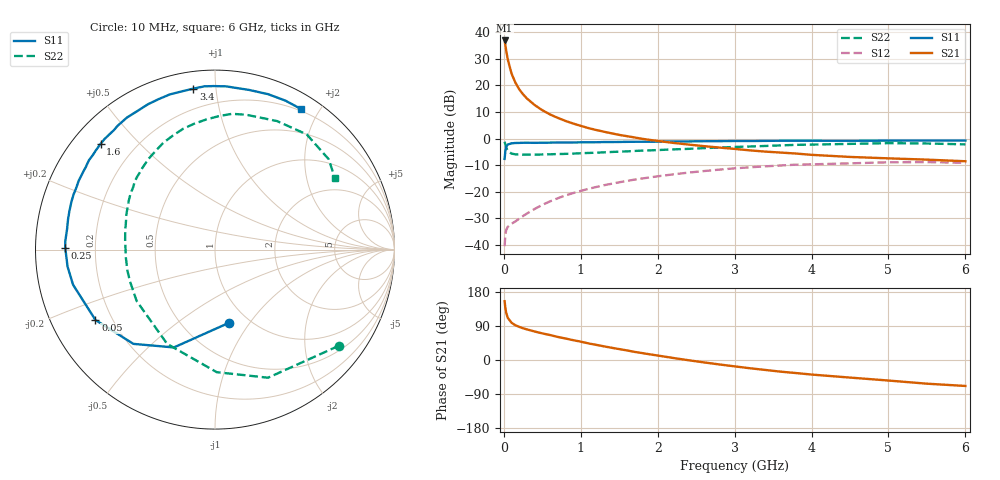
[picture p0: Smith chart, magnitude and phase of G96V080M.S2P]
! SIEMENS Small Signal Semiconductors
! BFG235
! Si NPN RF Bipolar Junction Transistor in SOT223
! VCE = 6 V  IC = 80 mA
! Common Emitter S-Parameters:  July  1994
# GHz  S  MA  R  50
!  f  S11  S21  S12  S22
! GHz  MAG  ANG  MAG  ANG  MAG  ANG  MAG  ANG
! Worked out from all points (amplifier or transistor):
!   40 points, 10 MHz to 6 GHz, reference 50 ohm
!   highest |S21| = 36.9 dB at 10 MHz (marker M1)
!   |S21| within 3 dB of that: start of sweep to 26.44 MHz
!   unconditionally stable (mu >= 1): 472 MHz to 1.295 GHz; 1.364 GHz to 1.405 GHz
!   at 200 MHz: K = 0.74, MSG = 24.3 dB, |S12| = -30.1 dB
!   at 1.5 GHz: K = 0.99, MSG = 8.9 dB, |S12| = -16.4 dB
!   at 6 GHz: K = 0.90, MSG = 0.3 dB, |S12| = -9.1 dB
!   S11 on the Smith chart (normalised r, x): 10 MHz: 0.82, -0.80; 50 MHz: 0.14, -0.27; 250 MHz: 0.09, +0.01; 1.6 GHz: 0.08, +0.39; 3.4 GHz: 0.09, +0.87; 6 GHz: 0.18, +1.76
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0.01  0.4152 -79.1  69.91 155.2  0.0095 67.0  0.873 -37.9
0.02  0.5913 -112.8  56.85 137.1  0.0157 52.2  0.7726 -67.5
0.03  0.6948 -130.9  45.84 125.1  0.0189 43.5  0.683 -89.2
0.05  0.7729 -149.5  31.23 111.6  0.0219 34.2  0.5891 -116.9
0.1  0.8147 -166.1  16.7 98.3  0.0251 33.9  0.5221 -146.7
0.15  0.8271 -173.5  11.27 91.7  0.0277 38.6  0.5056 -159.5
0.2  0.8292 -177.3  8.44 87.4  0.0313 42.6  0.5018 -166.7
0.25  0.8344 179.4  6.8 83.7  0.035 46.6  0.4986 -171.5
0.3  0.8355 176.8  5.676 80.8  0.039 49.2  0.4988 -175.4
0.4  0.832 172.2  4.275 75.2  0.0476 53.4  0.4987 179.2
0.5  0.836 168.3  3.413 70.2  0.0567 55.0  0.5028 174.9
0.6  0.8391 165.2  2.846 65.9  0.066 55.6  0.5066 171.0
0.7  0.8431 161.6  2.454 60.9  0.0755 55.8  0.5123 167.6
0.9  0.846 156.1  1.921 52.4  0.0945 53.9  0.5223 161.6
1.1  0.8525 149.7  1.575 43.8  0.1136 51.3  0.537 155.8
1.6  0.868 137.3  1.111 25.3  0.1598 42.1  0.5744 142.3
2.2  0.8843 123.7  0.831 5.4  0.2124 29.5  0.6266 126.3
3.2  0.9006 102.0  0.6 -21.8  0.2886 6.2  0.7102 99.6
3.4  0.905 97.7  0.569 -26.3  0.3007 1.4  0.7269 93.8
4.5  0.9097 77.9  0.452 -46.4  0.3426 -24.2  0.7951 64.3
5.5  0.918 64.7  0.402 -62.5  0.3611 -46.4  0.8093 38.5
6  0.9183 58.7  0.375 -68.5  0.3509 -54.7  0.7785 31.0
